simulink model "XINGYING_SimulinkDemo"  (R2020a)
settings: Solver=VariableStepAuto  StartTime=0.0  StopTime=1000.0  RelTol=1e-3
libraries: sldrtlib x1

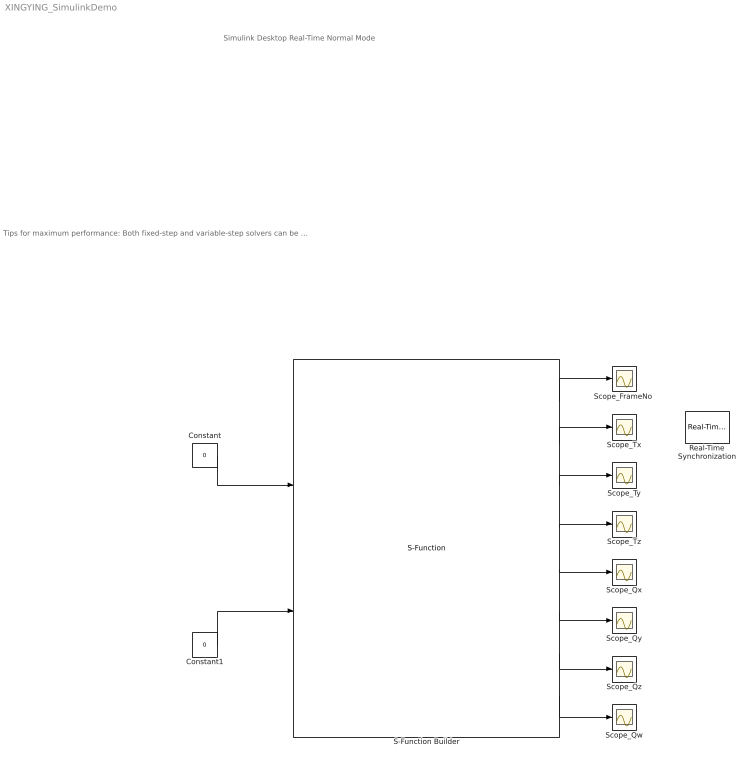
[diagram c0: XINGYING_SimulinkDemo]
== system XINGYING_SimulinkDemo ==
  note: Simulink Desktop Real-Time Normal Mode
  note: Tips for maximum performance: Both fixed-step and variable-step solvers can be used in Normal mode. All I/O blocks perform real-time synchronizaton. Use the Real-Time Synchronization block only if no I/O block is used. Use a single block that reads or writes all channels of given type, rather than multiple blocks for one channel each.
  Constant : Constant  Value=0  OutDataTypeStr=int32
  Constant1 : Constant  Value=0  OutDataTypeStr=int32
  Real-Time Synchronization : sldrtlib/Real-Time Synchronization  Commented=on  SampleTime=0.1  MaxMissedTicks=10  ShowMissedTicks=off  YieldWhenWaiting=off
  S-Function Builder : S-Function  InitFcn=try, set_param(gcb,'FunctionName','Get_Data_From_XINGYING_API'), end  FunctionName=Get_Data_From_XINGYING_API  SFunctionModules=Get_Data_From_XINGYING_API_wrapper  SFunctionDeploymentMode=off  EnableBusSupport=off  mask(S-Function Builder){}
      mask help: Simulink:masks:SFunctionBuilder_MD
      mask init:
      | val = [[.9  0.75 0.75 1 1 .9 .9 1]',[1 1 0.75 0.75 .9 .9 1 .9]'];try , sys = get_param(gcb,'SfunBuilderFcnName');if isempty(sys), sys = get_param(gcb,'FunctionName'); end,catch, sys = get_param(gcb,'FunctionName'); end
  "Scope_FrameNo " : Scope
  Scope_Qw : Scope
  Scope_Qx : Scope
  Scope_Qy : Scope
  Scope_Qz : Scope
  Scope_Tx : Scope
  Scope_Ty : Scope
  Scope_Tz : Scope
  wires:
  Constant/1 -> S-Function Builder/1
  Constant1/1 -> S-Function Builder/2
  S-Function Builder/1 -> "Scope_FrameNo "/1
  S-Function Builder/2 -> Scope_Tx/1
  S-Function Builder/3 -> Scope_Ty/1
  S-Function Builder/4 -> Scope_Tz/1
  S-Function Builder/5 -> Scope_Qx/1
  S-Function Builder/6 -> Scope_Qy/1
  S-Function Builder/7 -> Scope_Qz/1
  S-Function Builder/8 -> Scope_Qw/1
